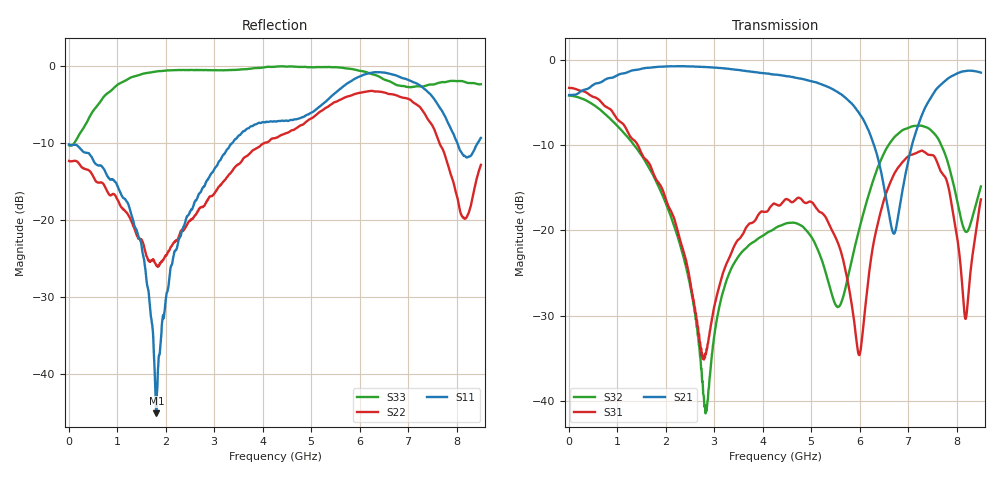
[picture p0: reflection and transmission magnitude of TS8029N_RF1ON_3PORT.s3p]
!Created with skrf (http://scikit-rf.org).
# GHz S RI R 50.0
!freq ReS11 ImS11 ReS12 ImS12 ReS13 ImS13
! ReS21 ImS21 ReS22 ImS22 ReS23 ImS23
! ReS31 ImS31 ReS32 ImS32 ReS33 ImS33
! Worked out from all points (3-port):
!   1601 points, 10 MHz to 8.5 GHz, reference 50 ohm
!   strongest paths, dB at 10 MHz, 2.132 GHz, 4.255 GHz, 6.378 GHz, 8.5 GHz:
!     S21: -4.1, -0.7, -1.7, -11.5, -1.5
!     S31: -3.3, -18.0, -16.9, -19.1, -16.4
!     S32: -4.2, -18.7, -19.8, -12.5, -14.8
!   lowest |S11| = -45.0 dB at 1.809 GHz (marker M1), VSWR 1.01, Z = 50.5 + j0.204 ohm
!   |S11| at or under -10 dB: start of sweep to 3.369 GHz; 8.016 GHz to 8.432 GHz (416 MHz wide, 5.06 % of centre)
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0.01  -0.3106 0.00501  0.6229 0.00142  0.6858 -0.00942
      0.6227 0.00131  -0.2427 0.0041  0.6184 -0.0097
      0.6858 -0.00948  0.6186 -0.0096  -0.3058 0.0158
1.24105  -0.0295 0.1209  0.8291 -0.2075  0.0429 -0.3651
         0.8285 -0.2075  0.031 0.102  0.00215 -0.346
         0.0429 -0.3645  0.00184 -0.3462  0.8157 0.1611
1.808819  0.00522 0.00202  0.791 -0.452  -0.0583 -0.1899
          0.7907 -0.452  0.0442 -0.025  -0.1107 -0.1579
          -0.0582 -0.1897  -0.1107 -0.1577  0.8399 -0.3814
2.827619  -0.1008 -0.1432  0.5004 -0.7594  0.012 -0.0146
          0.4999 -0.7591  -0.118 -0.0516  -0.0024 0.00843
          0.012 -0.0146  -0.0024 0.00843  0.2207 -0.917
4.255  -0.4054 -0.1671  -0.0682 -0.818  0.1058 -0.0967
       -0.0688 -0.8173  -0.3295 0.0874  0.0807 -0.0637
       0.1053 -0.0969  0.0809 -0.0636  -0.7297 -0.6692
5.990144  -0.7036 0.4854  -0.4186 -0.2515  -0.0161 0.00923
          -0.4184 -0.2513  0.00329 0.6711  0.0984 0.0242
          -0.0161 0.00927  0.0986 0.0241  -0.7196 0.5939
6.584444  -0.4253 0.7897  -0.1145 -0.0714  0.1681 0.0547
          -0.1143 -0.0716  0.443 0.4897  0.2962 -0.1023
          0.1679 0.0546  0.2958 -0.103  -0.1221 0.7942
7.884475  0.2374 0.308  -0.2663 -0.7541  -0.1036 -0.1072
          -0.2663 -0.7549  0.0448 -0.191  -0.1497 -0.1544
          -0.1036 -0.1069  -0.1492 -0.1539  0.8013 0.0349
8.186931  0.0814 0.2452  -0.5129 -0.6923  -0.00972 0.0287
          -0.5132 -0.6919  -0.0936 -0.0427  -0.0254 -0.095
          -0.00965 0.0287  -0.0255 -0.0949  0.5969 -0.5087
8.5  -0.0749 0.3342  -0.6561 -0.5291  0.1503 0.0221
     -0.6568 -0.5286  -0.1891 0.1288  0.0664 -0.1682
     0.1505 0.0217  0.0662 -0.1687  0.0144 -0.7627
